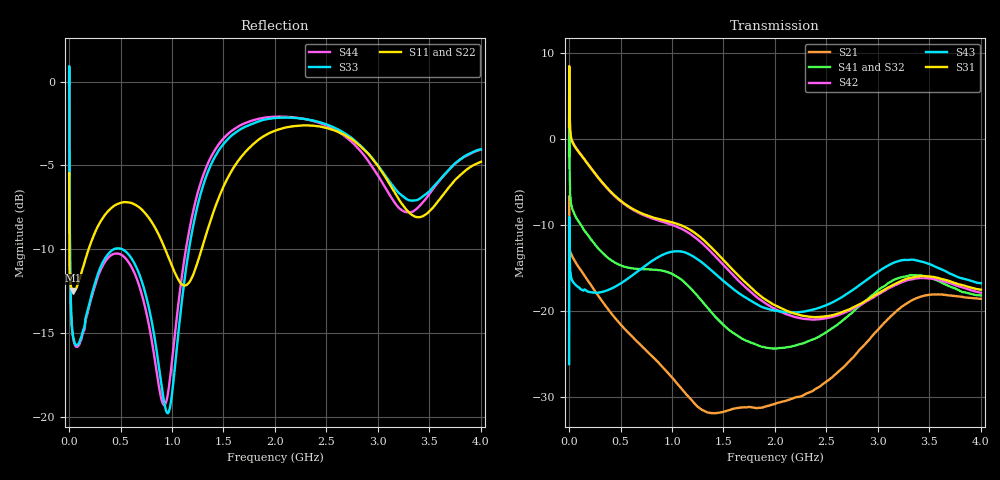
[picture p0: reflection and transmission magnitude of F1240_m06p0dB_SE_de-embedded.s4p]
! Integrated Device Technology
! Corporate Headquarters
! 6024 Silver Creek Valley Road
! San Jose, CA 95138  USA
! Phone:  1-408-284-8200
! Toll Free:  1-800-223-1366
! Webpage:  http://www.idt.com/
! Timing and RF Division
! 515 Groton Road, Suite 102
! Westford, MA 01886-6024
! Device:  F1240
! Description: Dual Intermediate Frequency Digital Variable Gain Amplifier
! Frequency:  10.0 -  500.00 MHz
! Package:  5x5 mm QFN Plastic Package: 32 pin
! Ports:  8 RF, 20 DC
!  Pin  1  = GA3 / Data  Pin 17  = RF OUT_B+
!  Pin  2  = GA4 / CLK  Pin 18  = RF OUT_B-
!  Pin  3  = GA5  Pin 19  = STBY_B
!  Pin  4  = VMODE  Pin 20  = Ground
!  Pin  5  = No Connect  Pin 21  = Ground
!  Pin  6  = GB5  Pin 22  = STB_A
!  Pin  7  = GB4  Pin 23  = RF OUT_A-  = Port 4
!  Pin  8  = GB3  Pin 24  = RF OUT_A+  = Port 3
!  Pin  9  = GB2  Pin 25  = GA0
!  Pin 10  = GB1  Pin 26  = ISET_A
!  Pin 11  = RF IN_B+  Pin 27  = VCC
!  Pin 12  = RF IN_B-  Pin 28  = Ground
!  Pin 13  = Ground  Pin 29  = RF IN_A-  = Port 2
!  Pin 14  = VCC  Pin 30  = RF IN_A+  = Port 1
!  Pin 15  = ISET_B  Pin 31  = GA1
!  Pin 16  = GB0  Pin 32  = GA2 / CSb
! Gain  = +19.5 dB
! State  = 1
! Voltage  = +5.00 V
! Current  = 85.292 mA (one channel only)
! Temperture  =  +25 C
! Test Date  =  2017-10-18
! Board  =  EB4031
! Data:  The device was measured on a custom evaluation board which has
!  individual transmission lines to the RF pins.  Data was collected
!  using a calibrated network analyzer.  The evaluation board was
!  de-embedded using Automatic Fixture Removal.
!  The reference plane is the edge of the package pin.
!  Only Channel A was measured.
!  This data is in single-ended operation.  If your needs are balanced
!  or differential S-parameters then this file needs to be used a
!  linear simulator.
! File Date:  2017-11-10  MJV
! Note:
!  Integrated Device Technology supplies this data as a sample of measured
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# Hz S dB R 100
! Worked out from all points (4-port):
!   410 points, 500 kHz to 4 GHz, reference 100 ohm
!   strongest paths, dB at 500 kHz, 930 MHz, 1.96 GHz, 2.98 GHz, 4 GHz:
!     S31: 1.4, -9.5, -19.0, -18.1, -17.5
!     S43: -26.1, -13.3, -19.8, -15.6, -16.7
!     S42: 1.4, -9.7, -19.5, -18.2, -17.9
!     S41: -2.0, -15.4, -24.3, -17.8, -18.2
!     S32: -2.0, -15.6, -24.2, -18.1, -18.6
!     S21: -6.7, -26.7, -30.9, -22.4, -18.6
!   lowest |S11| = -12.5 dB at 40 MHz (marker M1), VSWR 1.62, Z = 141 - j41 ohm
!   |S11| at or under -10 dB: 2.995 MHz to 189.5 MHz (186.5 MHz wide, 194 % of centre); 934 MHz to 1.288 GHz (353.5 MHz wide, 31.8 % of centre)
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500000  -5.51 -5.6  -6.70 -5.9  -31.25 78.6  -34.84 77.2
        -6.71 -5.8  -5.51 -5.6  -34.82 76.1  -31.23 79.8
        1.43 -109.9  -1.97 -111.9  -0.17 0.2  -26.11 -38.9
        -1.99 -110.8  1.43 -108.8  -26.12 -38.9  -0.18 2.5
2000000  -8.04 -30.2  -9.61 -30.8  -22.73 22.9  -27.03 5.6
         -9.61 -30.8  -8.02 -30.3  -26.98 5.4  -22.72 23.2
         7.81 177.8  3.80 162.1  -0.34 -52.5  -9.05 -142.4
         3.76 162.4  7.81 178.1  -9.04 -142.4  -0.38 -52.2
4000000  -10.89 -24.4  -12.37 -20.6  -23.42 5.9  -30.11 -12.8
         -12.37 -20.7  -10.89 -24.7  -30.08 -13.1  -23.40 6.0
         4.35 157.1  -1.83 140.1  -4.84 -84.8  -11.62 175.3
         -1.87 140.3  4.36 157.3  -11.62 175.2  -4.89 -84.8
4e7  -12.47 -35.1  -13.82 -20.6  -24.41 -13.8  -32.83 -16.9
     -13.83 -20.7  -12.45 -35.6  -32.84 -16.8  -24.36 -13.8
     -0.56 155.8  -8.39 146.7  -15.23 -157.2  -16.64 157.4
     -8.39 146.8  -0.50 155.7  -16.61 157.3  -15.30 -157.7
5.3e8  -7.19 -151.1  -21.91 -130.0  -27.93 -106.2  -36.36 -89.4
       -21.91 -129.8  -7.15 -152.1  -36.50 -87.3  -28.21 -106.3
       -7.44 24.0  -14.91 -27.7  -10.04 -174.2  -16.63 8.3
       -14.80 -29.0  -7.51 22.4  -16.55 8.1  -10.42 -174.8
2.89e9  -4.22 102.7  -23.64 -29.1  -27.85 -156.8  -30.08 -141.9
        -23.61 -29.1  -4.00 103.4  -30.74 -128.9  -29.24 -150.1
        -18.73 -70.8  -19.02 -152.7  -4.19 97.3  -17.18 -87.9
        -18.69 -164.0  -18.85 -67.6  -16.37 -85.7  -4.60 90.0
4e9  -4.78 -128.8  -18.56 116.2  -26.80 -32.7  -27.81 -17.2
     -18.55 116.2  -4.51 -127.5  -28.41 -2.7  -28.70 -23.8
     -17.50 47.3  -18.56 -51.0  -4.04 -133.4  -18.18 63.0
     -18.16 -65.3  -17.86 53.4  -16.75 56.1  -4.06 -143.3
